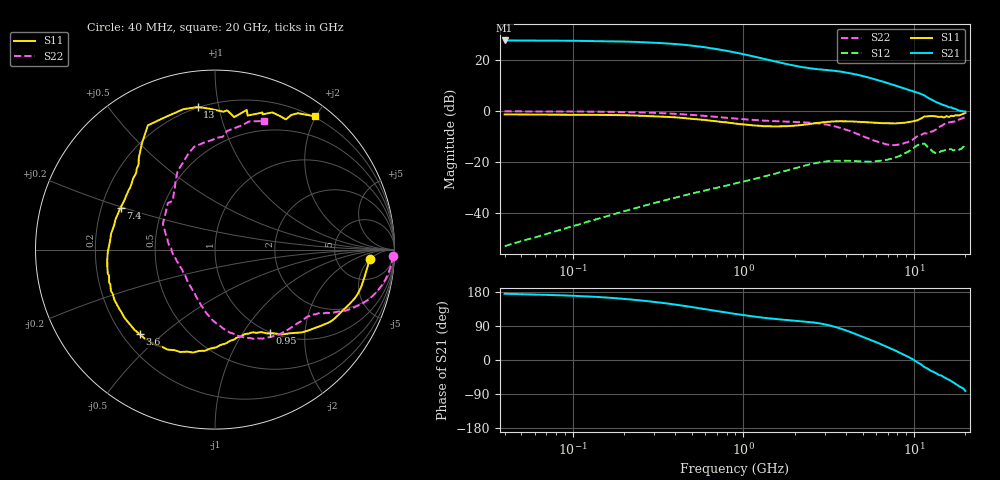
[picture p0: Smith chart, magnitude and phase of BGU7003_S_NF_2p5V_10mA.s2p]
!	Filename:	P:\Prog\Test\Noise\ATS_data\Testdata_Net\BGU7002	BGU7003	RN20082092\BGU7003_B1_high	freq_bias	loop_2.53V9.09mA_D.s2p
!	Date/Time:	Tue	16-Sep-08	9:23:53
!	BGU7003_B1_high	freq_bias	loop
!	bias	mode	1:00	Vout=	2.53	"V,"	Iout=	9.14	"mA,"	Vin=	4.146	"V,"	Iin=	0.9515	mA
!	Date/time	Mon	Aug	11	0:39:20	2008
!	Device	data	file	deembeded	for	feedlines	and	parallel
!	Original	file:	\BGU7002	BGU7003	RN20082092\BGU7003_B1_high	freq_bias	loop_2.53V9.09mA_R.s2p
!	Feed-files:	PR029V01_high	"frequency_140808_Feed1.s2p,"	PR029V01_high	frequency_140808_Feed2.s2p
!	Parallel-file:	PR029V01_high	frequency_140808_Par.s2p
#	MHz	S	MA	R	50
!	Freq-MHz	S11-mag	S11-arg	S21-mag	S21-arg	S12-mag	S12-arg	S22-mag	S22-arg
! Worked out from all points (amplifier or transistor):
!   156 points, 40 MHz to 20 GHz, reference 50 ohm
!   highest |S21| = 27.8 dB at 40 MHz (marker M1)
!   |S21| within 3 dB of that: start of sweep to 643.4 MHz
!   unconditionally stable (mu >= 1): nowhere
!   at 300 MHz: K = 0.26, MSG = 31.5 dB, |S12| = -36.1 dB
!   at 2.15 GHz: K = 0.60, MSG = 19.7 dB, |S12| = -21.9 dB
!   at 20 GHz: K = 0.31, MSG = 7.2 dB, |S12| = -14.5 dB
!   lowest NFmin = 0.57 dB at 400 MHz
!   S11 on the Smith chart (normalised r, x): 40 MHz: 12, -5; 950 MHz: 0.98, -1.33; 3.6 GHz: 0.27, -0.42; 7.4 GHz: 0.28, +0.20; 13 GHz: 0.20, +0.87; 20 GHz: 0.19, +1.98
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40  0.8626 -3.4  24.49 174.8  0.00222 76.3  0.9907 -2.0
80  0.8543 -7.0  24.24 171.2  0.00439 80.8  0.9867 -4.3
120  0.8469 -10.5  23.95 168.0  0.00658 81.1  0.9799 -6.5
190  0.8353 -16.4  23.43 162.2  0.01023 79.3  0.963 -10.2
230  0.8216 -19.7  23.01 158.8  0.01227 78.0  0.9501 -12.1
320  0.7829 -26.7  21.86 151.9  0.01653 75.2  0.9187 -16.0
410  0.7511 -32.9  20.7 145.5  0.0205 72.5  0.8808 -19.6
550  0.6857 -41.3  18.63 136.7  0.02593 69.4  0.8244 -23.6
700  0.6255 -48.2  16.55 129.1  0.03118 66.9  0.7687 -26.7
900  0.5668 -55.2  14.16 121.5  0.03781 64.8  0.7145 -29.5
950  0.5566 -56.9  13.65 120.0  0.03947 64.4  0.7056 -30.1
1150  0.5224 -62.0  11.85 114.8  0.046 62.8  0.6714 -32.1
1500  0.5004 -69.5  9.623 108.7  0.05789 59.6  0.6362 -35.9
1950  0.5145 -80.2  7.919 104.2  0.07356 54.1  0.6149 -42.2
2600  0.5715 -98.8  6.782 98.9  0.09386 43.5  0.585 -54.7
3600  0.6302 -131.5  6.058 84.8  0.1061 26.5  0.4803 -77.5
5000  0.6124 -167.2  4.917 61.3  0.1023 17.0  0.3246 -103.3
7200  0.5757 158.3  3.458 31.6  0.1139 19.0  0.2191 -143.5
7400  0.5756 156.0  3.355 29.2  0.1163 19.1  0.2147 -147.7
10500  0.6627 129.9  2.305 -6.5  0.2145 3.0  0.3244 153.5
13000  0.8007 96.9  1.612 -31.3  0.1564 -32.5  0.4071 123.4
20000  0.9272 53.2  0.9835 -81.8  0.1885 -60.8  0.7663 69.2
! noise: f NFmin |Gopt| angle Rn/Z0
400  0.568  0.247  10.04  0.123
1000  0.671  0.242  25.99  0.136
1500  0.756  0.24  39.28  0.141
1700  0.79  0.239  44.6  0.142
2200  0.876  0.24  57.89  0.142
3000  1.013  0.243  79.15  0.135
4400  1.252  0.259  116.4  0.114
5800  1.491  0.289  153.6  0.092
8000  1.867  0.361  -159.4  0.094
1.2e+04  2.551  0.575  -113.1  0.383
